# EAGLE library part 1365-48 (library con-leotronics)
DUAL ROW STRAIGHT HEADER 1364 SERIES. 1.27mm x 1.27mm. Without Fixing Post. SMT Source: http://www.leotronics.co.uk/Conexcon/Data%20Sheets/sec.%20A/1364ing.pdf
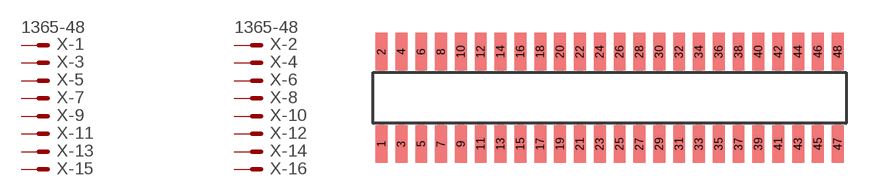
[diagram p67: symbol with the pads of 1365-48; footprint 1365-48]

Designator prefix X; gates -1=MVAL -2=MVAL -3=M -4=M -5=M -6=M -7=M -8=M -9=M -10=M -11=M -12=M -13=M -14=M -15=M -16=M -17=M -18=M -19=M -20=M -21=M -22=M -23=M -24=M -25=M -26=M -27=M -28=M -29=M -30=M -31=M -32=M -33=M -34=M -35=M -36=M -37=M -38=M -39=M -40=M -41=M -42=M -43=M -44=M -45=M -46=M -47=M -48=M

## 1365-48 (OC_FARNELL: unknown; OC_NEWARK: unknown)  [1365-48]
1  -1:S  pas
2  -2:S  pas
3  -3:S  pas
4  -4:S  pas
5  -5:S  pas
6  -6:S  pas
7  -7:S  pas
8  -8:S  pas
9  -9:S  pas
10  -10:S  pas
11  -11:S  pas
12  -12:S  pas
13  -13:S  pas
14  -14:S  pas
15  -15:S  pas
16  -16:S  pas
17  -17:S  pas
18  -18:S  pas
19  -19:S  pas
20  -20:S  pas
21  -21:S  pas
22  -22:S  pas
23  -23:S  pas
24  -24:S  pas
25  -25:S  pas
26  -26:S  pas
27  -27:S  pas
28  -28:S  pas
29  -29:S  pas
30  -30:S  pas
31  -31:S  pas
32  -32:S  pas
33  -33:S  pas
34  -34:S  pas
35  -35:S  pas
36  -36:S  pas
37  -37:S  pas
38  -38:S  pas
39  -39:S  pas
40  -40:S  pas
41  -41:S  pas
42  -42:S  pas
43  -43:S  pas
44  -44:S  pas
45  -45:S  pas
46  -46:S  pas
47  -47:S  pas
48  -48:S  pas

## Footprint 1365-48 (pad centres in mm)
DUAL ROW STRAIGHT HEADER 1364 SERIES. 1.27mm x 1.27mm. Without Fixing Post. SMT Source: http://www.leotronics.co.uk/Conexcon/Data%20Sheets/sec.%20A/1364ing.pdf
smd 0.76 x 2.4: 1 -14.605,-2.95; 2 -14.605,2.95; 3 -13.335,-2.95; 4 -13.335,2.95; 5 -12.065,-2.95; 6 -12.065,2.95; 7 -10.795,-2.95; 8 -10.795,2.95; 9 -9.525,-2.95; 10 -9.525,2.95; 11 -8.255,-2.95; 12 -8.255,2.95; 13 -6.985,-2.95; 14 -6.985,2.95; 15 -5.715,-2.95; 16 -5.715,2.95; 17 -4.445,-2.95; 18 -4.445,2.95; 19 -3.175,-2.95; 20 -3.175,2.95; 21 -1.905,-2.95; 22 -1.905,2.95; 23 -0.635,-2.95; 24 -0.635,2.95; 25 0.635,-2.95; 26 0.635,2.95; 27 1.905,-2.95; 28 1.905,2.95; 29 3.175,-2.95; 30 3.175,2.95; 31 4.445,-2.95; 32 4.445,2.95; 33 5.715,-2.95; 34 5.715,2.95; 35 6.985,-2.95; 36 6.985,2.95; 37 8.255,-2.95; 38 8.255,2.95; 39 9.525,-2.95; 40 9.525,2.95; 41 10.795,-2.95; 42 10.795,2.95; 43 12.065,-2.95; 44 12.065,2.95; 45 13.335,-2.95; 46 13.335,2.95; 47 14.605,-2.95; 48 14.605,2.95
